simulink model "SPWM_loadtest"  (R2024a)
settings: Solver=VariableStepAuto  StartTime=0.0  StopTime=1  FixedStep=1e-6  MaxStep=1e-5  RelTol=1e-2
libraries: spsIGBTDiodeLib x6, spsDiodeLib x6, spsThreePhaseSeriesRLCBranchLib x5, spsSeriesRLCBranchLib x3, spsThreePhaseVIMeasurementLib x3, spsGroundLib x3, spsThreePhaseBreakerLib x3, spsMultimeterLib x3, spsTHDLib x2, spsThreePhaseSourceLib x1, spsPVArrayLib x1, spsPower3phInstantaneousLib x1

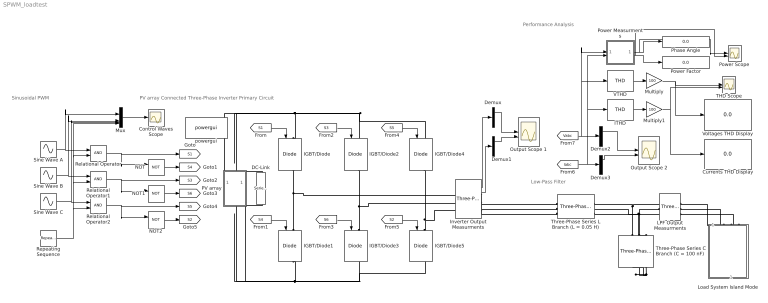
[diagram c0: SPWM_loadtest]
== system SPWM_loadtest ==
  note: Performance Analysis
  note: PV array Connected Three-Phase Inverter Primary Circuit
  note: Sinusoidal PWM
  note: Low-Pass Filter
  Control Waves Scope : Scope
  Currents THD Display : Display
  DC-Link : spsSeriesRLCBranchLib/Series RLC Branch  LConnTagsString=__new0  RConnTagsString=__new0  BranchType=RC  Resistance=20e-3  Inductance=1e-3  SetiL0=off  InitialCurrent=0  Capacitance=81e-6  Setx0=off  InitialVoltage=0  Measurements=None
  Demux{,1..3} (4 alike) : Demux  Outputs=3
  IGBT/Diode{,1..5} (6 alike) : spsIGBTDiodeLib/IGBT//Diode  Ron=1e-3  Rs=1e5  Cs=inf  Measurements=on
  ITHD : spsTHDLib/THD  Freq=50  Ts=0
  Inverter Output Measurments : spsThreePhaseVIMeasurementLib/Three-Phase V-I Measurement  VoltageMeasurement=phase-to-ground  SetLabelV=off  LabelV=Vabc  Vpu=off  VpuLL=off  CurrentMeasurement=yes  SetLabelI=off  LabelI=Iabc  Ipu=off  Pbase=100e6  Vbase=500e3  OutputType=Complex  PhasorSimulation=off  PSBequivalent=0
  LPF Output Measurments : spsThreePhaseVIMeasurementLib/Three-Phase V-I Measurement  VoltageMeasurement=phase-to-ground  SetLabelV=on  LabelV=Vabc  Vpu=off  VpuLL=off  CurrentMeasurement=yes  SetLabelI=on  LabelI=Iabc  Ipu=off  Pbase=100e6  Vbase=500e3  OutputType=Complex  PhasorSimulation=off  PSBequivalent=0
  Load System Island Mode : Subsystem
  Multiply : Gain  Gain=100
  Multiply1 : Gain  Gain=100
  Mux : Mux
  NOT : Logic  Operator=NOT  IconShape=distinctive  AllPortsSameDT=off  OutDataTypeStr=boolean
  NOT1 : Logic  Operator=NOT  IconShape=distinctive  AllPortsSameDT=off  OutDataTypeStr=boolean
  NOT2 : Logic  Operator=NOT  IconShape=distinctive  AllPortsSameDT=off  OutDataTypeStr=boolean
  Output Scope 1 : Scope  NumInputPorts=2
  Output Scope 2 : Scope  NumInputPorts=2
  PV array : Subsystem
  Phase Angle : Display
  Power Measurments : Subsystem
  Power Factor : Display
  Power Scope : Scope  NumInputPorts=2
  Relational Operator : RelationalOperator  OutDataTypeStr=boolean  RndMeth=Simplest
  Relational Operator1 : RelationalOperator  OutDataTypeStr=boolean  RndMeth=Simplest
  Relational Operator2 : RelationalOperator  OutDataTypeStr=boolean  RndMeth=Simplest
  Repeating Sequence : simulink/Sources/Repeating Sequence  rep_seq_t=[0 1 2 3]*[1/20000]  rep_seq_y=[0 1 -1 0]
  Sine Wave A : Sin  Frequency=100*pi  SampleTime=0
  Sine Wave B : Sin  Frequency=100*pi  Phase=2*pi/3  SampleTime=0
  Sine Wave C : Sin  Frequency=100*pi  Phase=-2*pi/3  SampleTime=0
  THD Scope : Scope  NumInputPorts=2
  Three-Phase Series C Branch (C = 100 nF) : spsThreePhaseSeriesRLCBranchLib/Three-Phase Series RLC Branch  LConnTagsString=A|B|C  RConnTagsString=A|B|C  BranchType=C  Resistance=1  Inductance=500e-6  Capacitance=100e-6  Measurements=None
  Three-Phase Series L Branch (L = 0.05 H) : spsThreePhaseSeriesRLCBranchLib/Three-Phase Series RLC Branch  LConnTagsString=A|B|C  RConnTagsString=A|B|C  BranchType=L  Resistance=1  Inductance=500e-4  Capacitance=1e-6  Measurements=None
  VTHD : spsTHDLib/THD  Freq=50  Ts=0
  Voltages THD Display : Display
  powergui : spspowerguiLib/powergui  Priority=1  SimulationMode=Continuous  SampleTime=1e-6  frequency=60  Iterations=50  frequencyindice=0  Pbase=100e6  ErrMax=1e-4  UnitsV=kV  UnitsW=MW  buscounter=0  FunctionMessages=off  echomessages=off  EnableUseOfTLC=off  CurrentSourceSwitches=off  DisableSnubberDevices=off  DisableRonSwitches=off  DisableVfSwitches=off  DisplayEquations=off  AutomaticDiscreteSolvers=off  SolverType=Tustin/Backward Euler (TBE)  Interpol=off  ExternalGateDelay=off  methode=off  Ts=100  x0status=blocks  SPID=on  SwTol=0  HookPort=off  NonlinearTolerance=1e-4  nMaxIteration=100  ContinueOnMaxIteration=off  RestoreLinks=warning  ResistiveCurrentMeasurement=off  Frange=[0:2:500]  Ylog=off  Xlog=on  ShowGrid=off  save=off  variable=ZData  structure=0  ZoomFFT=off  StartTime=0.0  cycles=1  DisplayStyle=1  fundamental=60  FreqAxis=off  MaxFrequency=1000  frequencyindicesteady=1  RmsSteady=1  display=off
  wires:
  Sine Wave A/1 -> Relational Operator/1, Mux/1
  Sine Wave B/1 -> Relational Operator1/1, Mux/2
  Sine Wave C/1 -> Relational Operator2/1, Mux/3
  Repeating Sequence/1 -> Relational Operator2/2, Relational Operator1/2, Relational Operator/2, Mux/4
  Mux/1 -> Control Waves Scope/1
  NOT/1 -> [S4]
  Relational Operator/1 -> [S1], NOT/1
  Relational Operator1/1 -> [S3], NOT1/1
  NOT1/1 -> [S6]
  NOT2/1 -> [S2]
  Relational Operator2/1 -> [S5], NOT2/1
  [S1] -> IGBT/Diode/1
  [S4] -> IGBT/Diode1/1
  [S3] -> IGBT/Diode2/1
  [S6] -> IGBT/Diode3/1
  [S5] -> IGBT/Diode4/1
  [S2] -> IGBT/Diode5/1
  Inverter Output Measurments/1 -> Demux/1
  Demux/1 -> Output Scope 1/1
  Inverter Output Measurments/2 -> Demux1/1
  Demux2/1 -> Output Scope 2/1
  Demux3/1 -> Output Scope 2/2
  [Vabc] -> Power Measurments/1(Vabc), VTHD/1, Demux2/1
  [Iabc] -> ITHD/1, Power Measurments/2(Iabc), Demux3/1
  VTHD/1 -> Multiply/1
  ITHD/1 -> Multiply1/1
  Multiply1/1 -> THD Scope/2, Currents THD Display/1
  Power Measurments/2(Out2) -> Power Factor/1, Power Scope/2
  Power Measurments/1(Out1) -> Phase Angle/1, Power Scope/1
  Multiply/1 -> Voltages THD Display/1, THD Scope/1
  Demux1/1 -> Output Scope 1/2
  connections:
  IGBT/Diode2/LConn1 -- IGBT/Diode4/LConn1 -- DC-Link/LConn1 -- PV array/LConn1 -- IGBT/Diode/LConn1
  IGBT/Diode1/RConn1 -- DC-Link/RConn1 -- PV array/RConn1 -- IGBT/Diode3/RConn1 -- IGBT/Diode5/RConn1
  IGBT/Diode5/LConn1 -- Inverter Output Measurments/LConn3 -- IGBT/Diode4/RConn1
  IGBT/Diode3/LConn1 -- IGBT/Diode2/RConn1 -- Inverter Output Measurments/LConn2
  IGBT/Diode1/LConn1 -- IGBT/Diode/RConn1 -- Inverter Output Measurments/LConn1
  Three-Phase Series C Branch (C = 100 nF)/RConn3 -- Three-Phase Series C Branch (C = 100 nF)/RConn1 -- Three-Phase Series C Branch (C = 100 nF)/RConn2
  Three-Phase Series C Branch (C = 100 nF)/LConn1 -- LPF Output Measurments/LConn1 -- Three-Phase Series L Branch (L = 0.05 H)/RConn1
  Three-Phase Series C Branch (C = 100 nF)/LConn2 -- Three-Phase Series L Branch (L = 0.05 H)/RConn2 -- LPF Output Measurments/LConn2
  Inverter Output Measurments/RConn1 -- Three-Phase Series L Branch (L = 0.05 H)/LConn1
  Inverter Output Measurments/RConn2 -- Three-Phase Series L Branch (L = 0.05 H)/LConn2
  Inverter Output Measurments/RConn3 -- Three-Phase Series L Branch (L = 0.05 H)/LConn3
  Three-Phase Series L Branch (L = 0.05 H)/RConn3 -- LPF Output Measurments/LConn3 -- Three-Phase Series C Branch (C = 100 nF)/LConn3
  LPF Output Measurments/RConn1 -- Load System Island Mode/LConn1
  LPF Output Measurments/RConn2 -- Load System Island Mode/LConn2
  LPF Output Measurments/RConn3 -- Load System Island Mode/LConn3

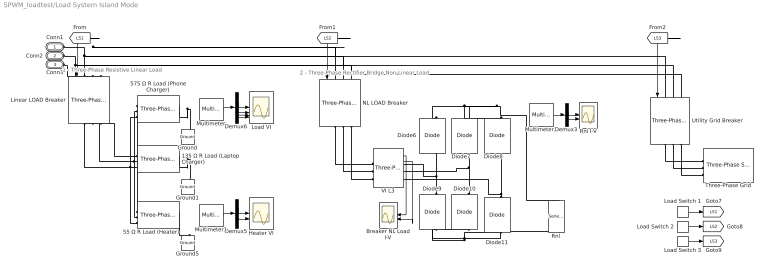
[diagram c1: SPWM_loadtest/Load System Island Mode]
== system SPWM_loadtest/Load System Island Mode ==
  note: 1 - Three-Phase Resistive Linear Load
  note: 2 - Three-Phase Rectifier Bridge Non-Linear Load
  135 Ω R Load (Laptop Charger) : spsThreePhaseSeriesRLCBranchLib/Three-Phase Series RLC Branch  LConnTagsString=A|B|C  RConnTagsString=A|B|C  BranchType=R  Resistance=135  Inductance=5.1e-3  Capacitance=1e-6  Measurements=Branch voltages and currents
  55 Ω R Load (Heater) : spsThreePhaseSeriesRLCBranchLib/Three-Phase Series RLC Branch  LConnTagsString=A|B|C  RConnTagsString=A|B|C  BranchType=R  Resistance=55  Inductance=5.1e-3  Capacitance=1e-6  Measurements=Branch voltages and currents
  575 Ω R Load (Phone Charger) : spsThreePhaseSeriesRLCBranchLib/Three-Phase Series RLC Branch  LConnTagsString=A|B|C  RConnTagsString=A|B|C  BranchType=R  Resistance=575  Inductance=5.1e-3  Capacitance=1e-6  Measurements=Branch voltages and currents
  Breaker NL Load I-V : Scope  NumInputPorts=2
  Demux3 : Demux  Outputs=2
  Demux5 : Demux  Outputs=2
  Demux6 : Demux
  Diode{6..11} (6 alike) : spsDiodeLib/Diode  Ron=0.001  Lon=0  Vf=0.8  IC=0  UseSnubber=0  Rs=10e+6  Cs=250e-9  Measurements=off
  Ground : spsGroundLib/Ground  LConnTagsString=a
  Ground1 : spsGroundLib/Ground  LConnTagsString=a
  Ground5 : spsGroundLib/Ground  LConnTagsString=a
  Heater VI : Scope  NumInputPorts=2
  Linear LOAD Breaker : spsThreePhaseBreakerLib/Three-Phase Breaker  InitialState=open  SwitchA=on  SwitchB=on  SwitchC=on  SwitchTimes="[1/60  5/60]"  External=on  BreakerResistance=0.01  SnubberResistance=1e6  SnubberCapacitance=inf  Measurements=None
  Load Switch 1 : DiscretePulseGenerator  PulseType=Time based  Period=3  PulseWidth=100/3
  Load Switch 2 : DiscretePulseGenerator  PulseType=Time based  Period=3  PulseWidth=100/3  PhaseDelay=1
  Load Switch 3 : DiscretePulseGenerator  PulseType=Time based  Period=3  PulseWidth=100/3  PhaseDelay=2
  Load VI : Scope  NumInputPorts=4
  Multimeter : spsMultimeterLib/Multimeter  L=20  sel=[8 2 18 12]  yselected={}  Gain=[1 1 1 1]  OutputType=Complex  PlotAtSimulationStop=off  PhasorSimulation=off
  Multimeter1 : spsMultimeterLib/Multimeter  L=20  sel=[5 15]  yselected={}  Gain=[1 1]  OutputType=Complex  PlotAtSimulationStop=off  PhasorSimulation=off
  Multimeter2 : spsMultimeterLib/Multimeter  L=20  sel=[1 11]  yselected={}  Gain=[1 1]  OutputType=Complex  PlotAtSimulationStop=off  PhasorSimulation=off
  NL LOAD Breaker : spsThreePhaseBreakerLib/Three-Phase Breaker  InitialState=open  SwitchA=on  SwitchB=on  SwitchC=on  SwitchTimes="[1/60  5/60]"  External=on  BreakerResistance=0.01  SnubberResistance=1e6  SnubberCapacitance=inf  Measurements=None
  Rnl : spsSeriesRLCBranchLib/Series RLC Branch  LConnTagsString=__new0  RConnTagsString=__new0  BranchType=R  Resistance=60  Inductance=1e-6  SetiL0=off  InitialCurrent=0  Capacitance=0.01598  Setx0=off  InitialVoltage=0  Measurements=Branch voltage and current
  Rnl I-V : Scope  NumInputPorts=2
  Three-Phase Grid : spsThreePhaseSourceLib/Three-Phase Source  InternalConnection=Yg  VoltagePhases=off  Voltage=340  PhaseAngle=0  Voltage_phases=[25e3 25e3 25e3]/sqrt(3)  PhaseAngles_phases=[0 -120 +120]  Frequency=50  NonIdealSource=on  SpecifyImpedance=off  Resistance=0.8929  Inductance=16.58e-3  ShortCircuitLevel=100e6  BaseVoltage=340  XRratio=7  BusType=swing  Pref=10e3  Qref=0  Prefabc=[10e3, 10e3, 10e3]  Qrefabc=[0, 0, 0]  Qmin=-inf  Qmax=inf
  Utility Grid Breaker : spsThreePhaseBreakerLib/Three-Phase Breaker  InitialState=open  SwitchA=on  SwitchB=on  SwitchC=on  SwitchTimes="[1/60  5/60]"  External=on  BreakerResistance=0.01  SnubberResistance=1e6  SnubberCapacitance=inf  Measurements=None
  VI L3 : spsThreePhaseVIMeasurementLib/Three-Phase V-I Measurement  VoltageMeasurement=phase-to-phase  SetLabelV=off  LabelV=Vabc  Vpu=off  VpuLL=off  CurrentMeasurement=yes  SetLabelI=off  LabelI=Iabc  Ipu=off  Pbase=100e6  Vbase=500e3  OutputType=Complex  PhasorSimulation=off  PSBequivalent=0
  Conn1 : PMIOPort  Side=Left
  Conn2 : PMIOPort  Port=2  Side=Left
  Conn3 : PMIOPort  Port=3  Side=Left
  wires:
  Demux5/2 -> Heater VI/2
  Demux6/2 -> Load VI/2
  Demux6/4 -> Load VI/4
  Demux6/1 -> Load VI/1
  Multimeter/1 -> Demux6/1
  Demux6/3 -> Load VI/3
  Demux5/1 -> Heater VI/1
  Multimeter1/1 -> Demux5/1
  Load Switch 3/1 -> [LS3]
  Load Switch 1/1 -> [LS1]
  Load Switch 2/1 -> [LS2]
  [LS1] -> Linear LOAD Breaker/1
  [LS2] -> NL LOAD Breaker/1
  [LS3] -> Utility Grid Breaker/1
  Multimeter2/1 -> Demux3/1
  Demux3/1 -> Rnl I-V/1
  Demux3/2 -> Rnl I-V/2
  VI L3/2 -> Breaker NL Load I-V/2
  VI L3/1 -> Breaker NL Load I-V/1
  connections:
  55 Ω R Load (Heater)/LConn2 -- 135 Ω R Load (Laptop Charger)/LConn2 -- Linear LOAD Breaker/RConn2 -- 575 Ω R Load (Phone Charger)/LConn2
  55 Ω R Load (Heater)/LConn3 -- 135 Ω R Load (Laptop Charger)/LConn3 -- Linear LOAD Breaker/RConn3 -- 575 Ω R Load (Phone Charger)/LConn3
  55 Ω R Load (Heater)/RConn1 -- 55 Ω R Load (Heater)/RConn2 -- 55 Ω R Load (Heater)/RConn3 -- Ground5/LConn1
  55 Ω R Load (Heater)/LConn1 -- 135 Ω R Load (Laptop Charger)/LConn1 -- Linear LOAD Breaker/RConn1 -- 575 Ω R Load (Phone Charger)/LConn1
  575 Ω R Load (Phone Charger)/RConn1 -- Ground/LConn1 -- 575 Ω R Load (Phone Charger)/RConn3 -- 575 Ω R Load (Phone Charger)/RConn2
  135 Ω R Load (Laptop Charger)/RConn1 -- Ground1/LConn1 -- 135 Ω R Load (Laptop Charger)/RConn3 -- 135 Ω R Load (Laptop Charger)/RConn2
  Utility Grid Breaker/RConn1 -- Three-Phase Grid/RConn1
  Utility Grid Breaker/RConn3 -- Three-Phase Grid/RConn3
  Utility Grid Breaker/RConn2 -- Three-Phase Grid/RConn2
  Conn1/RConn1 -- NL LOAD Breaker/LConn1 -- Utility Grid Breaker/LConn1 -- Linear LOAD Breaker/LConn1
  Conn2/RConn1 -- NL LOAD Breaker/LConn2 -- Utility Grid Breaker/LConn2 -- Linear LOAD Breaker/LConn2
  Conn3/RConn1 -- NL LOAD Breaker/LConn3 -- Utility Grid Breaker/LConn3 -- Linear LOAD Breaker/LConn3
  Rnl/LConn1 -- Diode8/RConn1 -- Diode6/RConn1 -- Diode7/RConn1
  Diode9/RConn1 -- VI L3/RConn1 -- Diode6/LConn1
  Diode11/RConn1 -- VI L3/RConn3 -- Diode8/LConn1
  Diode9/LConn1 -- Rnl/RConn1 -- Diode11/LConn1 -- Diode10/LConn1
  Diode7/LConn1 -- Diode10/RConn1 -- VI L3/RConn2
  NL LOAD Breaker/RConn1 -- VI L3/LConn1
  NL LOAD Breaker/RConn2 -- VI L3/LConn2
  NL LOAD Breaker/RConn3 -- VI L3/LConn3

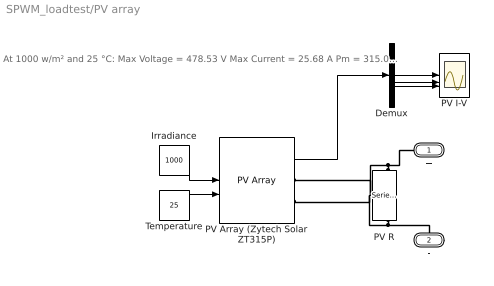
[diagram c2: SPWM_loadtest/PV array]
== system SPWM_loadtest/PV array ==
  note: At 1000 w/m² and 25 °C: Max Voltage = 478.53 V Max Current = 25.68 A Pm = 315.0936
  Demux : Demux  Outputs=5
  Irradiance : Constant  Value=1000
  PV I-V : Scope  NumInputPorts=5
  PV Array (Zytech Solar ZT315P) : spsPVArrayLib/PV Array  Npar=3  Nser=13  PlotType=array @ 25 deg.C & specified irradiances  S_vec="[ 1000  500  100 ]"  Temp_C_vec="[ 45 25  ]"  ModuleName=Zytech Solar ZT315P  PlotWhenSelected=off  Pm=315.0936  Ncell=72  Voc=46.44  Isc=9.01  Vm=36.81  Im=8.56  beta_Voc_pc=-0.3199  alpha_Isc_pc=0.048302  beta_Voc=-0.14856  alpha_Isc=0.004352  IL=9.0792  I0=6.901e-11  nI=0.9809  Rsh=572.7811  Rs=0.50125  RobustModel=off  RobustCellTemperature=313.3991  BAL=on  Tc=1e-6  Tfilter=5e-5
  PV R : spsSeriesRLCBranchLib/Series RLC Branch  LConnTagsString=__new0  RConnTagsString=__new0  BranchType=R  Resistance=17.2  Inductance=1e-3  SetiL0=off  InitialCurrent=0  Capacitance=1e-6  Setx0=off  InitialVoltage=0  Measurements=None
  Temperature : Constant  Value=25
  + : PMIOPort  Side=Left
  - : PMIOPort  Port=2  Side=Right
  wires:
  Irradiance/1 -> PV Array (Zytech Solar ZT315P)/1
  Temperature/1 -> PV Array (Zytech Solar ZT315P)/2
  PV Array (Zytech Solar ZT315P)/1 -> Demux/1
  Demux/3 -> PV I-V/3
  Demux/2 -> PV I-V/2
  Demux/1 -> PV I-V/1
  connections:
  PV R/LConn1 -- +/RConn1 -- PV Array (Zytech Solar ZT315P)/RConn1
  PV R/RConn1 -- -/RConn1 -- PV Array (Zytech Solar ZT315P)/RConn2

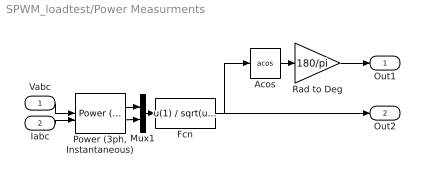
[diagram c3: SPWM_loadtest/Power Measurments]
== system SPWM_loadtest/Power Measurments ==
  Vabc : Inport
  Iabc : Inport  Port=2
  Acos : Trigonometry  Operator=acos
  Fcn : Fcn  Expr=u(1) / sqrt(u(1)^2 + u(2)^2)
  Mux1 : Mux  Inputs=2
  "Power (3ph, Instantaneous)" : spsPower3phInstantaneousLib/Power (3ph, Instantaneous)
  Rad to Deg : Gain  Gain=180/pi
  Out1 : Outport
  Out2 : Outport  Port=2
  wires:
  "Power (3ph, Instantaneous)"/2 -> Mux1/2
  Acos/1 -> Rad to Deg/1
  Fcn/1 -> Out2/1, Acos/1
  Vabc/1 -> "Power (3ph, Instantaneous)"/1
  Iabc/1 -> "Power (3ph, Instantaneous)"/2
  Mux1/1 -> Fcn/1
  "Power (3ph, Instantaneous)"/1 -> Mux1/1
  Rad to Deg/1 -> Out1/1
